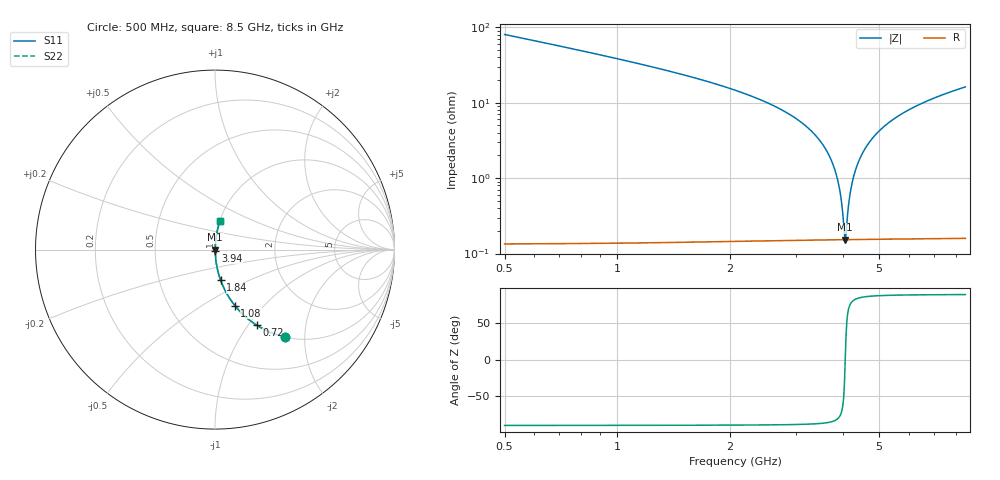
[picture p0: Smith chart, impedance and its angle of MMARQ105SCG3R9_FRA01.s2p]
! MMARQ105SCG3R9_FRA01  S-PARAMETER MODEL  ( General Type )
! Model Generated by TAIYO YUDEN Corporation (http://www.ty-top.com)
! Version 1.0
! TAIYO YUDEN Control No. 200326
! Copyright(c) 2020 TAIYO YUDEN CO.,LTD. All Rights Reserved.
! Product Description (link to TY-COMPAS)
! https://ds.yuden.co.jp/TYCOMPAS/or/detail?pn=MMARQ105SCG3R9BFRA01&u=M
! Products Name : Multilayer Ceramic Capacitors
! Characteristics :
!  Capacitance : 3.9 pF , Rated Voltage : 250V , TCC : CG / C0G
!  Case Size : 1.0 x 0.5 / 0.039 x 0.02 [mm/inch] , Thickness : 0.5 / 0.02 [mm/inch]
!  (Conditions: Temperature = 25 degC , DC Bias Current/Voltage = 0A / 0V)
! External Node Assignments :
!  1  o---| |---o  2
! GND o---------o GND
! Frequency Range : 500MHz  -  8.5GHz  [ 401 STEP ]
# MHz S RI R 50
! Freq[MHz].  S11 Real  S11 Imag  S21 Real  S21 Imag  S12 Real  S12 Imag  S22 Real  S22 Imag
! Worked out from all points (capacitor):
!   401 points, 500 MHz to 8.5 GHz, reference 50 ohm
!   read as one part in series: C = 3.9 pF near 540 MHz
!   lowest |Z| = 153 mohm at 4.06 GHz (marker M1)
!   series resonance near 4.06 GHz, so ESL is about 390 pH
!   S11 on the Smith chart (normalised r, x): 500 MHz: 1.00, -1.61; 720 MHz: 1.00, -1.10; 1.08 GHz: 1.00, -0.70; 1.84 GHz: 1.00, -0.35; 3.94 GHz: 1.00, -0.01; 8.5 GHz: 1.00, +0.32
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500  0.3928 -0.4875  0.6072 0.4875  0.6072 0.4875  0.3928 -0.4875
720  0.2322 -0.421  0.7678 0.421  0.7678 0.421  0.2322 -0.421
1080  0.1107 -0.3118  0.8893 0.3118  0.8893 0.3118  0.1107 -0.3118
1840  0.0314 -0.1704  0.9686 0.1704  0.9686 0.1704  0.0314 -0.1704
2660  0.00905 -0.0866  0.9909 0.0866  0.9909 0.0866  0.00905 -0.0866
3180  0.00394 -0.0493  0.9961 0.0493  0.9961 0.0493  0.00394 -0.0493
3460  0.00255 -0.0321  0.9975 0.0321  0.9975 0.0321  0.00255 -0.0321
3680  0.00191 -0.0197  0.9981 0.0197  0.9981 0.0197  0.00191 -0.0197
3840  0.00165 -0.0112  0.9984 0.0112  0.9984 0.0112  0.00165 -0.0112
3940  0.00156 -0.00601  0.9984 0.00601  0.9984 0.00601  0.00156 -0.00601
4020  0.00153 -0.00198  0.9985 0.00198  0.9985 0.00198  0.00153 -0.00198
4060  0.00153 -1.03e-06  0.9985 1.03e-06  0.9985 1.03e-06  0.00153 -1.03e-06
4080  0.00153 0.000983  0.9985 -0.000983  0.9985 -0.000983  0.00153 0.000983
4160  0.00155 0.00487  0.9984 -0.00487  0.9984 -0.00487  0.00155 0.00487
4240  0.00161 0.00869  0.9984 -0.00869  0.9984 -0.00869  0.00161 0.00869
4360  0.00174 0.0143  0.9983 -0.0143  0.9983 -0.0143  0.00174 0.0143
4500  0.00196 0.0206  0.998 -0.0206  0.998 -0.0206  0.00196 0.0206
4720  0.00246 0.0303  0.9975 -0.0303  0.9975 -0.0303  0.00246 0.0303
5020  0.00338 0.0428  0.9966 -0.0428  0.9966 -0.0428  0.00338 0.0428
5840  0.00708 0.074  0.9929 -0.074  0.9929 -0.074  0.00708 0.074
7180  0.0159 0.1187  0.9841 -0.1187  0.9841 -0.1187  0.0159 0.1187
8500  0.0271 0.1577  0.9729 -0.1577  0.9729 -0.1577  0.0271 0.1577
